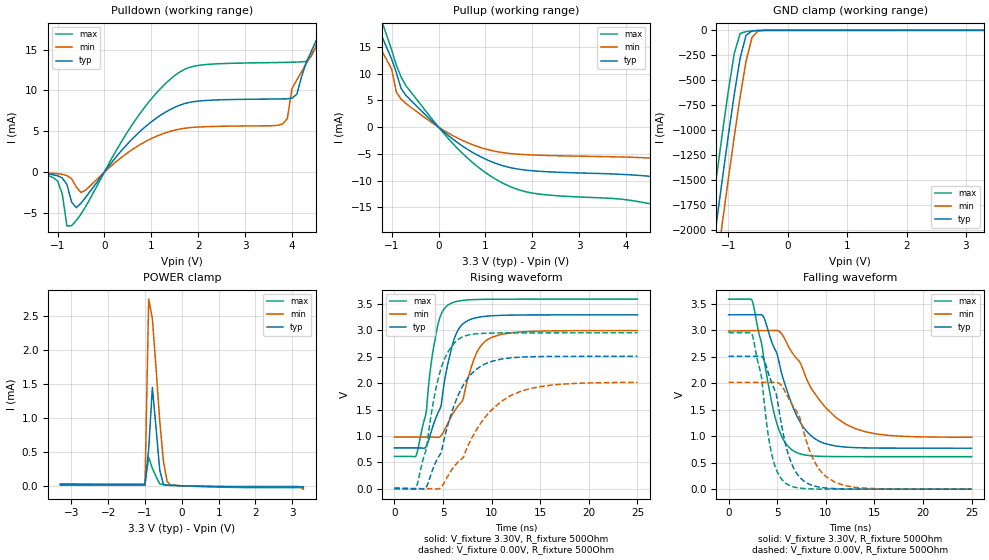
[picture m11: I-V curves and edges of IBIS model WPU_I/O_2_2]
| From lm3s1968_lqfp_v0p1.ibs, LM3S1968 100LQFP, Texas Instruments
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[Model]   WPU_I/O_2_2
Model_type   I/O
Vinl = 1.26
Vinh = 2.04
Vmeas = 1.65
| variable   typ   min   max
C_comp   9.739pF   9.739pF   9.739pF
[Model Spec]
Vinh+   1.91   1.78   2.04
Vinh-   1.90   1.76   2.03
Vinl+   1.40   1.27   1.54
Vinl-   1.39   1.26   1.53
| variable   typ   min   max
[Temperature Range]  25   85   -40
[Voltage Range]   3.3V   3.0V   3.6V
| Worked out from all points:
|   slope of the pulldown table from 0 to 0.495 V, typ, clamps not added: 143 ohm
|   slope of the pullup table from 0 to 0.495 V, typ, clamps not added: 143 ohm
|   GND clamp passes 1 mA (typ) near -0.48 V on its own axis
|   POWER clamp passes 1 mA (typ) near -0.73 V on its own axis
|   falling waveform, V_fixture 3.30V, R_fixture 500Ohm: 20-80 % time 2.91ns typ, 4.35ns min, 1.96ns max; typ from 3.29 V to 0.774 V
|   rising waveform, V_fixture 3.30V, R_fixture 500Ohm: 20-80 % time 1.93ns typ, 2.62ns min, 1.41ns max; typ from 0.774 V to 3.3 V
|   falling waveform, V_fixture 0.00V, R_fixture 500Ohm: 20-80 % time 2ns typ, 2.73ns min, 1.46ns max; typ from 2.51 V to 0 V
|   rising waveform, V_fixture 0.00V, R_fixture 500Ohm: 20-80 % time 2.98ns typ, 4.63ns min, 1.95ns max; typ from 0.002 V to 2.51 V
[Pulldown]
|  Voltage   I(typ)   I(min)   I(max)
-3.3V     -63.97uA   -36.29uA   -90.89uA
-1.1V     -317.2uA   -146.3uA   -639.6uA
-700mV    -3.674mA   -802.3uA   -6.561mA
-500mV    -3.8mA     -2.497mA   -5.141mA
600mV     4.106mA    2.793mA    5.879mA
1.5V      7.937mA    5.14mA     11.83mA
3.8V      8.962mA    5.903mA    13.43mA
4.1V      9.518mA    11.26mA    13.48mA
4.6V      17.2mA     16.24mA    17.2mA
4.8V      19.76mA    18.22mA    20.43mA
6.5V      43.78mA    32.33mA    51.9mA
6.6V      45.47mA    7.61mA     54.43mA
[Pullup]
|  Voltage   I(typ)   I(min)   I(max)
-3.3V     58.76mA    44.69mA    74.9mA
-1.5V     22.87mA    18.92mA    27.05mA
-1.3V     18.86mA    15.72mA    22.09mA
-1.2V     16.83mA    14.11mA    19.57mA
-1V       12.74mA    10.89mA    14.48mA
-900mV    10.18mA    6.552mA    11.57mA
-600mV    5.084mA    3.776mA    6.691mA
500mV     -3.481mA   -2.455mA   -4.825mA
1.5V      -7.517mA   -4.915mA   -11.03mA
5V        -9.793mA   -6.102mA   -15.25mA
5.9V      -11.98mA   -7.296mA   -18.76mA
6.6V      -15.07mA   -8.994mA   -23.96mA
[GND Clamp]
|  Voltage   I(typ)   I(min)   I(max)
-3.3V     -11.72A    -12.12A    -11.3A
-1.4V     -2.845A    -3.285A    -2.387A
-1.3V     -2.39A     -2.831A    -1.93A
-1.2V     -1.938A    -2.38A     -1.478A
-1.1V     -1.494A    -1.934A    -1.036A
-1V       -1.059A    -1.496A    -610.6mA
-900mV    -645mA     -1.069A    -232.9mA
-800mV    -277.1mA   -664.4mA   -31.6mA
-700mV    -48.56mA   -306.6mA   -12.11mA
-600mV    -5.565mA   -70.2mA    -6.295mA
-500mV    -1.181mA   -7.883mA   -2.191mA
3.3V      2.282nA    6.919uA    -6.845uA
[POWER Clamp]
|  Voltage   I(typ)   I(min)   I(max)
-3.3V     15.18uA    8.315uA    27.48uA
-1V       14.14uA    7.74uA     25.63uA
-900mV    539.2uA    2.746mA    419.4uA
-800mV    1.446mA    2.463mA    255uA
-700mV    851uA      1.726mA    135.8uA
-600mV    231.3uA    957.3uA    27.23uA
-500mV    21.69uA    361.2uA    14.14uA
-400mV    7.764uA    63.51uA    10.49uA
-300mV    5.5uA      6.919uA    7.727uA
3.1V      -16.64uA   -9.947uA   -27.43uA
3.2V      -16.65uA   -12.11uA   -27.44uA
3.3V      -16.65uA   -49.87uA   -27.45uA
[Ramp]
| variable   typ   min   max
dV/dt_f   1.51/2.91n   1.20/4.35n   1.79/1.96n
dV/dt_r   1.50/2.98n   1.20/4.63n   1.77/1.95n
R_load = 500Ohm
[Falling Waveform]
V_fixture = 3.30V
V_fixture_min = 3.00V
V_fixture_max = 3.60V
R_fixture = 500Ohm
|   Time   V(typ)   V(min)   V(max)
0s        3.294V     2.987V     3.591V
2.4ns     3.295V     2.994V     3.572V
3.6ns     3.254V     2.996V     2.513V
4.8ns     2.631V     2.997V     1.352V
5.6ns     2.098V     2.897V     949.6mV
6.6ns     1.561V     2.564V     732.8mV
8.9ns     951.9mV    1.8V       625.2mV
11ns      815.4mV    1.358V     615.6mV
13ns      784.7mV    1.146V     614.4mV
25ns      774.3mV    980.8mV    614.1mV
[Rising Waveform]
V_fixture = 3.30V
V_fixture_min = 3.00V
V_fixture_max = 3.60V
R_fixture = 500Ohm
|   Time   V(typ)   V(min)   V(max)
0s        774.3mV    980mV      614.1mV
2.3ns     774.3mV    980mV      662.6mV
3.3ns     811.2mV    979.9mV    1.493V
3.7ns     1.031V     979.9mV    2.265V
4.4ns     1.404V     973.1mV    3.047V
5.6ns     2.451V     1.283V     3.492V
6.9ns     3.097V     1.645V     3.566V
8.4ns     3.24V      2.553V     3.586V
9.9ns     3.277V     2.86V      3.59V
25ns      3.296V     2.998V     3.594V
[Falling Waveform]
V_fixture = 0.00V
V_fixture_min = 0.00V
V_fixture_max = 0.00V
R_fixture = 500Ohm
|   Time   V(typ)   V(min)   V(max)
0s        2.51V      2.018V     2.956V
2.4ns     2.51V      2.018V     2.935V
3.4ns     2.508V     2.018V     2.101V
4ns       2.248V     2.018V     1.126V
4.5ns     1.983V     2.019V     614.7mV
6ns       749.6mV    1.778V     97.34mV
7.7ns     161.8mV    1.102V     13.05mV
9.1ns     47.3mV     438.1mV    2.734mV
11ns      9.464mV    125mV      429.7uV
25ns      28.08uV    64.98uV    19.55uV
[Rising Waveform]
V_fixture = 0.00V
V_fixture_min = 0.00V
V_fixture_max = 0.00V
R_fixture = 500Ohm
|   Time   V(typ)   V(min)   V(max)
0s        2.15mV     21.53mV    118.1uV
2.2ns     361.2uV    5.668mV    6.533mV
3.2ns     10.4mV     3.135mV    701.8mV
4ns       395.4mV    2.151mV    1.641V
4.7ns     652.8mV    11.9mV     2.22V
5.5ns     1.212V     242.1mV    2.589V
6.7ns     1.829V     533.4mV    2.847V
8.7ns     2.298V     1.195V     2.94V
12ns      2.482V     1.769V     2.954V
25ns      2.51V      2.016V     2.955V
